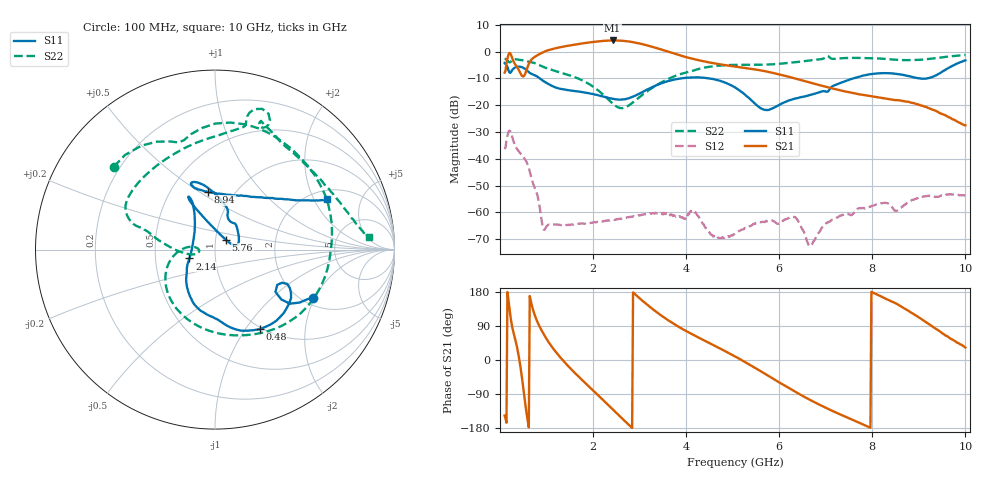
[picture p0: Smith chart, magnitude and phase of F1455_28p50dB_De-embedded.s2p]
! Integrated Device Technology
! Corporate Headquarters
! 6024 Silver Creek Valley Road
! San Jose, CA 95138  USA
! Phone:  1-408-284-8200
! Toll Free:  1-800-223-1366
! Webpage:  http://www.idt.com/
! Timing and RF Division
! 515 Groton Road, Suite 102
! Westford, MA 01886-6024
! Device:  F1455
! Description: 6-bit 0.5 dB Transmit Variable Gain Amplifier
! Frequency:  1400.0 -  2300.00 MHz
! Package:  6x6 mm Thin QFN Plastic Package: 28 pin
! State:  57
! Atten State:  28.5 dB
! Voltage:  +5.00 Volts
! Current:  217.614 mA
! Data:  The device was measured on a the F1455 evaluation board which has
!  individual transmission lines to the RF pins.  Data was collected
!  using a calibrated network analyzer.  The evaluation board was
!  de-embedded using a TRL calibration technique.
!  The reference plane is the edge of the package pin.
!  Pin  1 = CSb
!  Pin  2 = DATA
!  Pin  3 = CLK
!  Pin  4 = RSET
!  Pin  5 = GND
!  Pin  6 = RFIN  = Port 1
!  Pin  7 = GND
!  Pin  8 = NC
!  Pin  9 = NC
!  Pin 10 = NC
!  Pin 11 = NC
!  Pin 12 = NC
!  Pin 13 = NC
!  Pin 14 = /STBY
!  Pin 15 = GND
!  Pin 16 = RFOUT  = Port 2
!  Pin 17 = GND
!  Pin 18 = NC
!  Pin 19 = NC
!  Pin 20 = NC
!  Pin 21 = GND
!  Pin 22 = NC
!  Pin 23 = GND
!  Pin 24 = NC
!  Pin 25 = NC
!  Pin 26 = NC
!  Pin 27 = GND
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# GHz S dB R 50
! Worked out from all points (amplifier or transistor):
!   496 points, 100 MHz to 10 GHz, reference 50 ohm
!   highest |S21| = 4.1 dB at 2.42 GHz (marker M1)
!   |S21| within 3 dB of that: 1.175 GHz to 3.396 GHz (2.222 GHz wide, 97.2 % of centre)
!   unconditionally stable (mu >= 1): start of sweep to end of sweep
!   at 1.74 GHz: K = 507.62, MAG = 3.5 dB, |S12| = -64.2 dB
!   at 5.06 GHz: K = 1521.50, MAG = -3.7 dB, |S12| = -67.8 dB
!   at 10 GHz: K = 775.59, MAG = -18.8 dB, |S12| = -53.7 dB
!   S11 on the Smith chart (normalised r, x): 100 MHz: 2.27, -1.94; 480 MHz: 0.97, -1.17; 2.14 GHz: 0.75, -0.08; 5.76 GHz: 1.12, +0.12; 8.94 GHz: 0.76, +0.54; 10 GHz: 2.43, +2.55
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0.1  -4.29 -26.1  -7.86 -146.7  -36.38 47.7  -2.75 140.7
0.18  -6.70 -36.9  -1.27 161.4  -30.12 -6.4  -3.72 112.4
0.26  -6.99 -25.4  -2.27 89.1  -31.62 -77.3  -3.33 96.1
0.38  -5.66 -42.7  -6.11 25.9  -36.65 -118.6  -2.99 58.2
0.48  -5.88 -60.7  -9.18 -53.3  -38.84 -150.5  -3.25 31.7
0.66  -8.19 -87.9  -3.37 156.9  -46.05 139.7  -3.94 -10.1
0.8  -9.32 -105.7  -1.42 101.9  -53.31 108.2  -4.67 -41.1
0.96  -11.29 -123.6  0.00 64.0  -66.41 130.3  -5.92 -70.5
1.34  -14.03 -142.4  1.77 0.9  -64.58 119.7  -8.03 -120.9
1.76  -15.09 -151.1  2.99 -52.2  -64.06 90.0  -10.67 -157.6
2.14  -16.45 -161.0  3.85 -96.7  -63.41 76.0  -14.89 178.8
2.42  -17.61 -177.0  4.13 -129.9  -62.80 66.8  -19.37 173.4
2.82  -17.09 146.5  3.61 -177.1  -61.58 56.0  -19.47 -167.2
3.4  -12.30 118.5  1.11 123.3  -60.19 34.7  -12.20 177.2
4.08  -9.68 116.1  -2.45 71.2  -59.82 20.5  -7.45 163.5
5.06  -13.48 111.9  -5.61 8.8  -67.79 40.9  -4.97 148.6
5.76  -21.78 41.7  -7.55 -41.4  -63.13 32.0  -4.84 119.2
6.34  -17.54 14.1  -10.02 -83.5  -61.73 -10.7  -3.99 89.7
6.7  -16.09 34.3  -11.74 -107.7  -71.90 -173.7  -3.25 78.7
8.36  -8.08 109.5  -17.78 157.7  -56.83 65.4  -2.84 62.8
8.94  -9.80 97.0  -19.57 117.5  -54.91 76.9  -3.16 39.2
10  -3.30 24.1  -27.51 32.9  -53.68 9.4  -1.28 4.7
